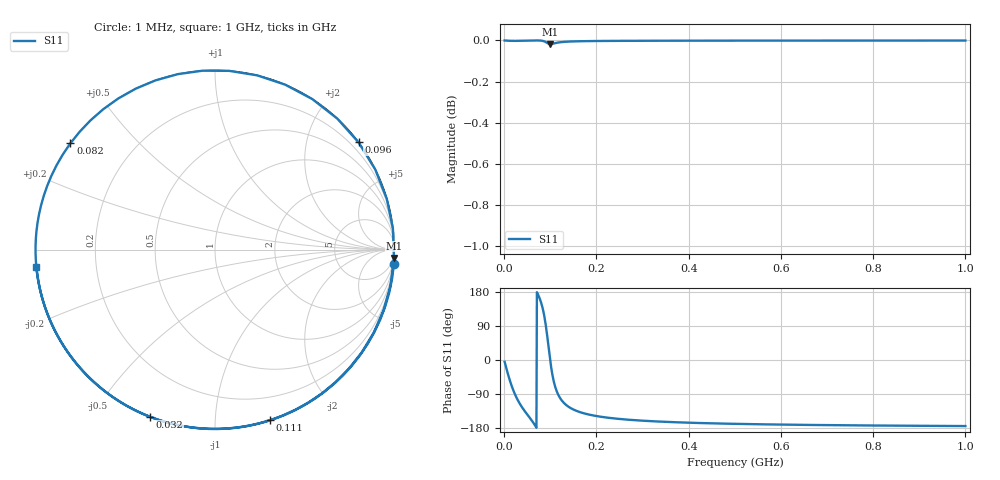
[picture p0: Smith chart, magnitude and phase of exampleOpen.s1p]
# MHz S RI R 50.0
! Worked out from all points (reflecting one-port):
!   999 points, 1 MHz to 1 GHz, reference 50 ohm
!   lowest |S11| = 0.0 dB at 100 MHz (marker M1), VSWR 983.20, Z = 93.4 - j2.14e+03 ohm
!   phase of S11 starts at -5 deg and turns -530 deg over the sweep
!   S11 on the Smith chart (normalised r, x): 1 MHz: 0, -25; 32 MHz: 0.00, -0.68; 82 MHz: 0.00, +0.33; 96 MHz: 0.01, +3.01; 111 MHz: 0.00, -1.38; 1 GHz: 0.00, -0.05
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1  0.9967 -0.0808
7  0.8499 -0.5266
16  0.3865 -0.922
23  0.0138 -0.9997
32  -0.3631 -0.9315
46  -0.7336 -0.6794
62  -0.9575 -0.2883
74  -0.9886 0.1502
82  -0.8053 0.5926
86  -0.5387 0.842
90  -0.0694 0.9967
93  0.3906 0.9191
96  0.7998 0.5974
100  0.9969 -0.0465
105  0.7462 -0.6629
108  0.5188 -0.853
111  0.308 -0.9498
118  -0.06 -0.9971
126  -0.3159 -0.9479
141  -0.5665 -0.8233
164  -0.736 -0.6763
251  -0.9112 -0.4115
376  -0.9633 -0.2678
502  -0.9799 -0.1989
626  -0.9872 -0.1589
751  -0.9912 -0.1322
876  -0.9935 -0.1132
1000  -0.995 -0.0991
